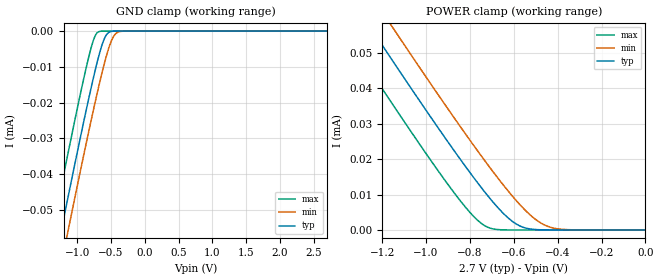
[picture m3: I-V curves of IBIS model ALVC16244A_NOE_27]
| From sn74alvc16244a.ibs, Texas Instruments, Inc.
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[Model]   ALVC16244A_NOE_27
Model_type  Input
Vinl=0.7
Vinh=1.7
| variable   typ   min   max
C_comp   0.78pF   0.51pF   0.95pF
[Temperature Range]   40   100   -40
| Ambient temperature   25   85   -40
[Voltage range]   2.7   2.7   2.7
[GND Clamp]
| ALVC16244A_NOE_27
|   Voltage   I(typ)   I(min)   I(max)
-2.7V     -195.6uA   -204.7uA   -183.8uA
-1.38V    -69.12uA   -78.54uA   -56.87uA
-1.24V    -55.98uA   -65.42uA   -43.69uA
-1.125V   -45.29uA   -54.73uA   -32.99uA
-825mV    -18.36uA   -27.57uA   -6.799uA
-750mV    -12.13uA   -21.09uA   -1.96uA
-690mV    -7.545uA   -16.08uA   -248.1nA
-620mV    -3.098uA   -10.58uA   -9.302nA
-560mV    -819.8nA   -6.351uA   -512pA
-470mV    -42.07nA   -1.73uA    -12.88pA
-375mV    -1.378nA   -157.4nA   -6.257pA
2.7V      5.11pA     7.205pA    4.886pA
[POWER Clamp]
| ALVC16244A_NOE_27
|   Voltage   I(typ)   I(min)   I(max)
-2.7V     195.6uA    204.7uA    183.8uA
-1.415V   72.42uA    81.84uA    60.18uA
-1.355V   66.76uA    76.19uA    54.51uA
-1.245V   56.45uA    65.89uA    44.16uA
-1.15V    47.61uA    57.05uA    35.31uA
-915mV    26.21uA    35.56uA    14.14uA
-780mV    14.58uA    23.65uA    3.647uA
-705mV    8.645uA    17.32uA    462.5nA
-595mV    1.93uA     8.747uA    2.773nA
-505mV    143.8nA    3.188uA    41.51pA
-420mV    6.982nA    547nA      6.911pA
-35.59fV  5.11pA     7.205pA    4.886pA
